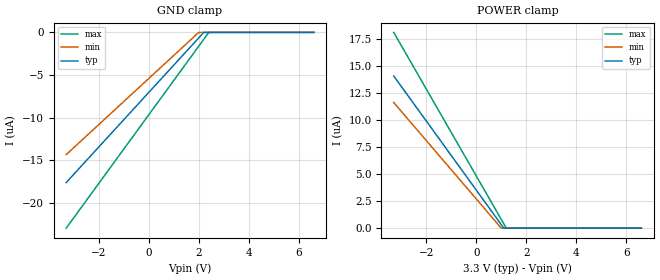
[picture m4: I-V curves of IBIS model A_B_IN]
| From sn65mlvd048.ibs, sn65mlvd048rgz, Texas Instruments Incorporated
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|   A_B Model
[Model]   A_B_IN
Model_type   Input
|Signals   B   negative pin
Vinl   = 0.8V
Vinh   = 2V
|To run as single ended tie second pin to 1.2V
|Common mode can be anywhere between -1V to 3.4V with Vdiff of over 50mV
|Rref_Diff   = 50Ohms
|C_comp   typ   min   max
|   (Nom PVT)   (Fast PVT)   (Slow PVT)
C_comp   2.5213736pF  2.2265813pF  2.7902078pF
[Voltage Range]   3.3   3.0   3.6
|Junction temperature
[Temperature Range]   37   97   -40
|ambient temperature   25   85   -40
[GND Clamp]
|   Voltage   I(typ)   I(min)   I(max)
-3.3V     -17.61uA   -14.33uA   -22.95uA
1.973V    -725.6nA   -71.99nA   -1.718uA
2.172V    -88.46nA   0A         -916.7nA
2.371V    0A         0A         -115.3nA
2.421V    0A         0A         0A
6.6V      0A         0A         0A
[POWER Clamp]
|   Voltage   I(typ)   I(min)   I(max)
-3.3V     14.09uA    11.63uA    18.12uA
978.4mV   389.4nA    58.54nA    892.5nA
1.078V    70.86nA    0A         491.8nA
1.177V    0A         0A         91.13nA
1.227V    0A         0A         0A
6.6V      0A         0A         0A
